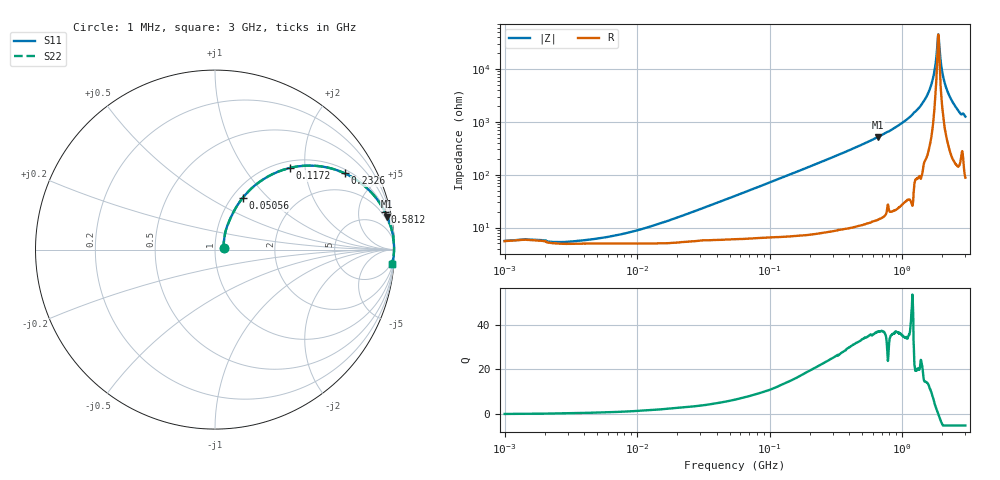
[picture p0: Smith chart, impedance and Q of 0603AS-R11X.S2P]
!s-Parameter Generated by FASTRON Sdn. Bhd.
!FASTRON P/N : 0603AS-R11X
!Keysight Technologies: E4991B_MY54100416_A.01.15
!Date created: Wed Oct 04 13:25:11 2023
!Version  : Rev01 Wed Oct 04 13:25:11 2023
!Data & Calibration Information:
!Freq	S11	S21	S12	S22
!PortZ  Port1:50+j0  Port2:50+j0
!When reading reference impedance value at option line is always used.
! Remarks : This data is being provided solely for informational purposes.
# Hz S dB R 50
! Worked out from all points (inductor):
!   1601 points, 1 MHz to 3 GHz, reference 50 ohm
!   read as one part in series: L = 115 nH near 22.03 MHz
!   highest Q = 36.9 at 658.6 MHz (marker M1), where L = 125 nH
!   self-resonance near 1.874 GHz
!   S11 on the Smith chart (normalised r, x): 1 MHz: 1.11, +0.01; 50.56 MHz: 1.12, +0.72; 117.2 MHz: 1.13, +1.66; 232.6 MHz: 1.15, +3.30; 581.2 MHz: 1.25, +8.88; 3 GHz: 3, -25
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1000000  -25.55 7.2  -0.47 -0.4  -0.47 -0.4  -25.55 7.2
3804036  -25.33 27.9  -0.42 -1.5  -0.42 -1.5  -25.33 27.9
1.447069e7  -19.14 58.8  -0.47 -5.7  -0.47 -5.7  -19.14 58.8
5.055795e7  -9.70 61.8  -0.98 -18.8  -0.98 -18.8  -9.70 61.8
5.477226e7  -9.11 61.0  -1.06 -20.3  -1.06 -20.3  -9.11 61.0
1.171891e8  -4.21 47.6  -2.61 -37.9  -2.61 -37.9  -4.21 47.6
2.083556e8  -1.83 33.2  -5.23 -54.0  -5.23 -54.0  -1.83 33.2
2.326032e8  -1.53 30.4  -5.90 -56.9  -5.90 -56.9  -1.53 30.4
5.81181e8  -0.27 12.6  -13.22 -75.8  -13.22 -75.8  -0.27 12.6
6.586299e8  -0.20 10.9  -14.50 -77.6  -14.50 -77.6  -0.20 10.9
7.925923e8  -0.14 8.6  -16.51 -79.5  -16.51 -79.5  -0.14 8.6
1.142072e9  -0.05 4.6  -21.84 -83.8  -21.84 -83.8  -0.05 4.6
1.488926e9  -0.03 2.1  -28.61 -83.9  -28.61 -83.9  -0.03 2.1
1.67892e9  -0.02 1.0  -34.95 -82.6  -34.95 -82.6  -0.02 1.0
1.747494e9  -0.02 0.6  -38.86 -78.8  -38.86 -78.8  -0.02 0.6
1.827992e9  -0.02 0.2  -46.57 -62.0  -46.57 -62.0  -0.02 0.2
1.874306e9  -0.02 0.0  -53.07 -1.9  -53.07 -1.9  -0.02 0.0
1.921792e9  -0.02 -0.2  -46.69 60.9  -46.69 60.9  -0.02 -0.2
2.050964e9  -0.02 -0.8  -36.52 79.4  -36.52 79.4  -0.02 -0.8
2.210833e9  -0.03 -1.6  -31.23 82.3  -31.23 82.3  -0.03 -1.6
2.660507e9  -0.06 -3.5  -24.18 81.3  -24.18 81.3  -0.06 -3.5
3e9  -0.08 -4.5  -22.05 81.5  -22.05 81.5  -0.08 -4.5
